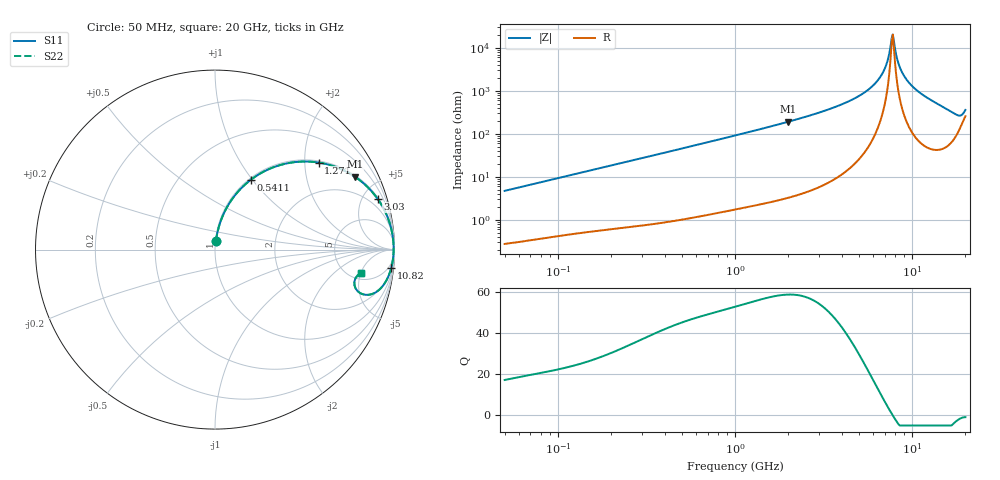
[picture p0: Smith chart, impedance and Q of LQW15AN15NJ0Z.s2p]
!Murata Part Number: LQW15AN15NJ0Z
!These Parameters are Measured in Series Mode Connection
!  o--[Z]--o
!Port1  Port2
!  o-------o
!Freq. Start=50[MHz] Stop=20[GHz], 401[Steps]
# Hz S RI R 50
!Freq.(Hz) S11(Real) S11(Imag) S21(Real) S21(Imag) S12(Real) S12(Imag) S22(Real) S22(Imag)
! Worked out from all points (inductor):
!   401 points, 50 MHz to 20 GHz, reference 50 ohm
!   read as one part in series: L = 15 nH near 51.52 MHz
!   highest Q = 58.6 at 1.992 GHz (marker M1), where L = 15.2 nH
!   self-resonance near 7.668 GHz
!   S11 on the Smith chart (normalised r, x): 50 MHz: 1.01, +0.09; 541.1 MHz: 1.02, +0.99; 1.271 GHz: 1.04, +2.35; 3.03 GHz: 1.12, +6.37; 10.82 GHz: 2, -19; 20 GHz: 6.16, -5.03
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5e7  0.00497 0.0469  0.995 -0.0469  0.995 -0.0469  0.00497 0.0469
1.364002e8  0.0204 0.1229  0.9796 -0.1229  0.9796 -0.1229  0.0204 0.1229
3.721004e8  0.1092 0.2998  0.8908 -0.2998  0.8908 -0.2998  0.1092 0.2998
5.411141e8  0.2007 0.3898  0.7993 -0.3898  0.7993 -0.3898  0.2007 0.3898
1e9  0.4571 0.4887  0.5429 -0.4887  0.5429 -0.4887  0.4571 0.4887
1.270815e9  0.5778 0.4849  0.4222 -0.4849  0.4222 -0.4849  0.5778 0.4849
1.99176e9  0.7805 0.4055  0.2195 -0.4055  0.2195 -0.4055  0.7805 0.4055
2.728004e9  0.8809 0.3151  0.1191 -0.3151  0.1191 -0.3151  0.8809 0.3151
3.029571e9  0.906 0.2827  0.094 -0.2827  0.094 -0.2827  0.906 0.2827
4.472136e9  0.9682 0.1623  0.0318 -0.1623  0.0318 -0.1623  0.9682 0.1623
5.856089e9  0.9888 0.0821  0.0112 -0.0821  0.0112 -0.0821  0.9888 0.0821
6.802353e9  0.994 0.0385  0.00598 -0.0385  0.00598 -0.0385  0.994 0.0385
7.114996e9  0.9948 0.0254  0.00522 -0.0254  0.00522 -0.0254  0.9948 0.0254
7.442007e9  0.9952 0.0124  0.00483 -0.0124  0.00483 -0.0124  0.9952 0.0124
7.668323e9  0.9952 0.00362  0.00477 -0.00362  0.00477 -0.00362  0.9952 0.00362
7.784049e9  0.9952 -0.000754  0.00481 0.000754  0.00481 0.000754  0.9952 -0.000754
7.901521e9  0.9951 -0.00514  0.00489 0.00514  0.00489 0.00514  0.9951 -0.00514
8.389408e9  0.9944 -0.0228  0.00562 0.0228  0.00562 0.0228  0.9944 -0.0228
8.774992e9  0.9934 -0.0361  0.00665 0.0361  0.00665 0.0361  0.9934 -0.0361
1.082228e10  0.9824 -0.1003  0.0176 0.1003  0.0176 0.1003  0.9824 -0.1003
1.721783e10  0.8494 -0.2521  0.1506 0.2521  0.1506 0.2521  0.8494 -0.2521
2e10  0.8129 -0.1314  0.1871 0.1314  0.1871 0.1314  0.8129 -0.1314
